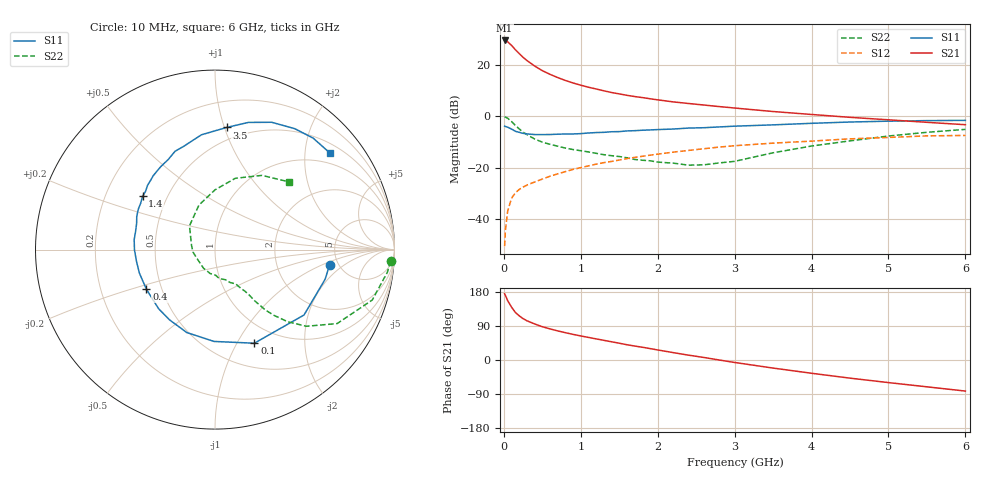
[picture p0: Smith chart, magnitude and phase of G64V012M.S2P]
! SIEMENS Small Signal Semiconductors
! BFG193
! Si NPN RF Bipolar Junction Transistor in SOT223
! VCE = 4 V  IC = 12 mA
! Common Emitter S-Parameters:  August  1996
# GHz  S  MA  R  50
!  f  S11  S21  S12  S22
! GHz  MAG  ANG  MAG  ANG  MAG  ANG  MAG  ANG
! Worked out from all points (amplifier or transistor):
!   36 points, 10 MHz to 6 GHz, reference 50 ohm
!   highest |S21| = 29.7 dB at 10 MHz (marker M1)
!   |S21| within 3 dB of that: start of sweep to 131.5 MHz
!   unconditionally stable (mu >= 1): 827 MHz to 2.49 GHz
!   at 250 MHz: K = 0.59, MSG = 25.4 dB, |S12| = -27.6 dB
!   at 1.4 GHz: K = 1.06, MAG = 12.0 dB, |S12| = -17.6 dB
!   at 6 GHz: K = 0.87, MSG = 2.1 dB, |S12| = -7.4 dB
!   S11 on the Smith chart (normalised r, x): 10 MHz: 4.25, -1.22; 100 MHz: 0.77, -1.18; 400 MHz: 0.41, -0.23; 1.4 GHz: 0.36, +0.29; 3.5 GHz: 0.40, +1.02; 6 GHz: 0.71, +2.56
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0.01  0.6443 -7.5  30.56 174.9  0.0029 90.4  0.9799 -3.7
0.02  0.6356 -15.0  30.4 170.8  0.0059 82.8  0.9691 -7.4
0.05  0.6154 -36.3  28.68 156.5  0.0141 74.5  0.9199 -17.8
0.1  0.5658 -67.2  24.5 139.6  0.025 64.6  0.7956 -31.2
0.15  0.5117 -90.6  20.11 125.5  0.0321 57.0  0.6646 -40.0
0.2  0.4881 -108.8  16.91 116.6  0.0373 54.5  0.5701 -44.8
0.25  0.4662 -123.0  14.32 109.2  0.0415 52.9  0.492 -48.1
0.3  0.4552 -133.6  12.39 103.5  0.0453 52.8  0.4408 -50.1
0.4  0.4415 -149.9  9.671 95.2  0.0522 52.9  0.3617 -52.2
0.5  0.4412 -162.8  7.851 87.8  0.0595 53.1  0.3138 -53.1
0.6  0.4423 -171.5  6.647 82.1  0.0676 53.6  0.2848 -54.3
0.7  0.4486 -179.7  5.754 76.8  0.0752 53.7  0.2616 -56.1
0.9  0.4538 167.2  4.508 67.6  0.0919 53.0  0.2249 -58.8
1.1  0.4737 157.0  3.721 59.6  0.1078 51.8  0.202 -65.2
1.4  0.5012 143.6  2.931 48.1  0.1316 47.9  0.1704 -75.2
1.7  0.5261 133.2  2.446 36.9  0.1577 43.5  0.1441 -87.9
2.2  0.566 117.3  1.924 19.6  0.2 34.0  0.122 -121.6
2.8  0.6226 101.1  1.556 0.0  0.2512 21.8  0.1231 -173.4
3.5  0.6834 84.6  1.246 -21.3  0.3001 5.6  0.1942 137.1
4.5  0.7765 66.0  0.959 -47.9  0.3639 -14.2  0.3325 90.1
5.5  0.8276 48.6  0.766 -70.8  0.4162 -38.2  0.4891 57.7
6  0.8361 40.2  0.688 -82.0  0.4244 -52.1  0.5576 42.7
